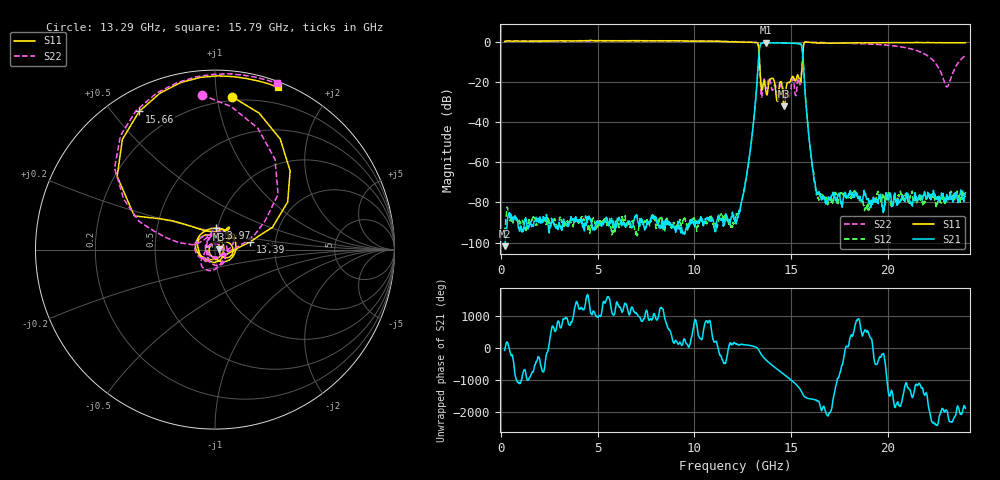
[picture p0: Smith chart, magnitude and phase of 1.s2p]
!Agilent Technologies,N5235A,US52150107,A.09.80.20
!Agilent N5235A: A.09.80.20
!Date: Tuesday, September 27, 2011 16:04:44
!Correction: S11(Full 2 Port(1,2))
!S21(Full 2 Port(1,2))
!S12(Full 2 Port(1,2))
!S22(Full 2 Port(1,2))
!S2P File: Measurements: S11, S21, S12, S22:
# Hz S  dB  R 50
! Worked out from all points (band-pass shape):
!   1601 points, 200 MHz to 24 GHz, reference 50 ohm
!   highest |S21| = -0.65 dB at 13.71 GHz (marker M1); lowest = -101.7 dB at 200 MHz (marker M2)
!   |S21| within 3 dB of the highest: 13.37 GHz to 15.56 GHz (2.195 GHz wide, 15.2 % of centre)
!   lowest |S11| = -32.2 dB at 14.64 GHz (marker M3), VSWR 1.05, Z = 52.5 + j0.289 ohm
!   |S11| at or under -10 dB: 13.37 GHz to 15.59 GHz (2.22 GHz wide, 15.3 % of centre)
!   |S22| runs from -29.5 to 0.4 dB; largest |S21 - S12| = 0.05
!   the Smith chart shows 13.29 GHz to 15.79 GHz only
!   S11 on the Smith chart (normalised r, x): 13.29 GHz: 0.17, +1.11; 13.39 GHz: 1.48, +0.13; 13.97 GHz: 0.98, +0.24; 15.66 GHz: 0.09, +0.59; 15.79 GHz: 0.05, +1.46
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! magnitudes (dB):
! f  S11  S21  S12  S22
! 200 MHz  0.0  -101.7  -95.1  0.0
! 4.172 GHz  0.4  -90.3  -87.2  0.2
! 8.143 GHz  0.4  -90.8  -88.3  0.4
! 12.1 GHz  -0.2  -89.5  -88.5  -0.1
! 12.41 GHz  -0.3  -80.6  -80.9  -0.1
! 12.65 GHz  -0.4  -69.7  -69.0  -0.1
! 13.01 GHz  -0.5  -44.7  -44.8  -0.2
! 13.29 GHz  -1.3  -12.6  -12.5  -1.3
! 13.39 GHz  -13.9  -2.1  -2.0  -15.8
! 13.71 GHz  -25.2  -0.6  -0.6  -23.2
! 13.97 GHz  -18.5  -0.7  -0.6  -22.4
! 14.64 GHz  -32.2  -0.8  -0.7  -27.3
! 15.37 GHz  -17.4  -1.1  -1.0  -18.6
! 15.52 GHz  -17.7  -1.5  -1.6  -17.9
! 15.66 GHz  -1.1  -14.8  -13.9  -1.0
! 15.79 GHz  -0.3  -33.7  -33.9  -0.1
! 16.07 GHz  -0.6  -60.3  -59.4  -0.3
! 16.41 GHz  -0.8  -75.8  -78.2  -0.5
! 20.04 GHz  -0.5  -78.6  -76.7  -1.9
! 22.05 GHz  -0.5  -77.2  -75.0  -7.2
! 23.05 GHz  -0.6  -76.1  -79.2  -22.6
! 24 GHz  -0.6  -75.2  -77.2  -7.0
